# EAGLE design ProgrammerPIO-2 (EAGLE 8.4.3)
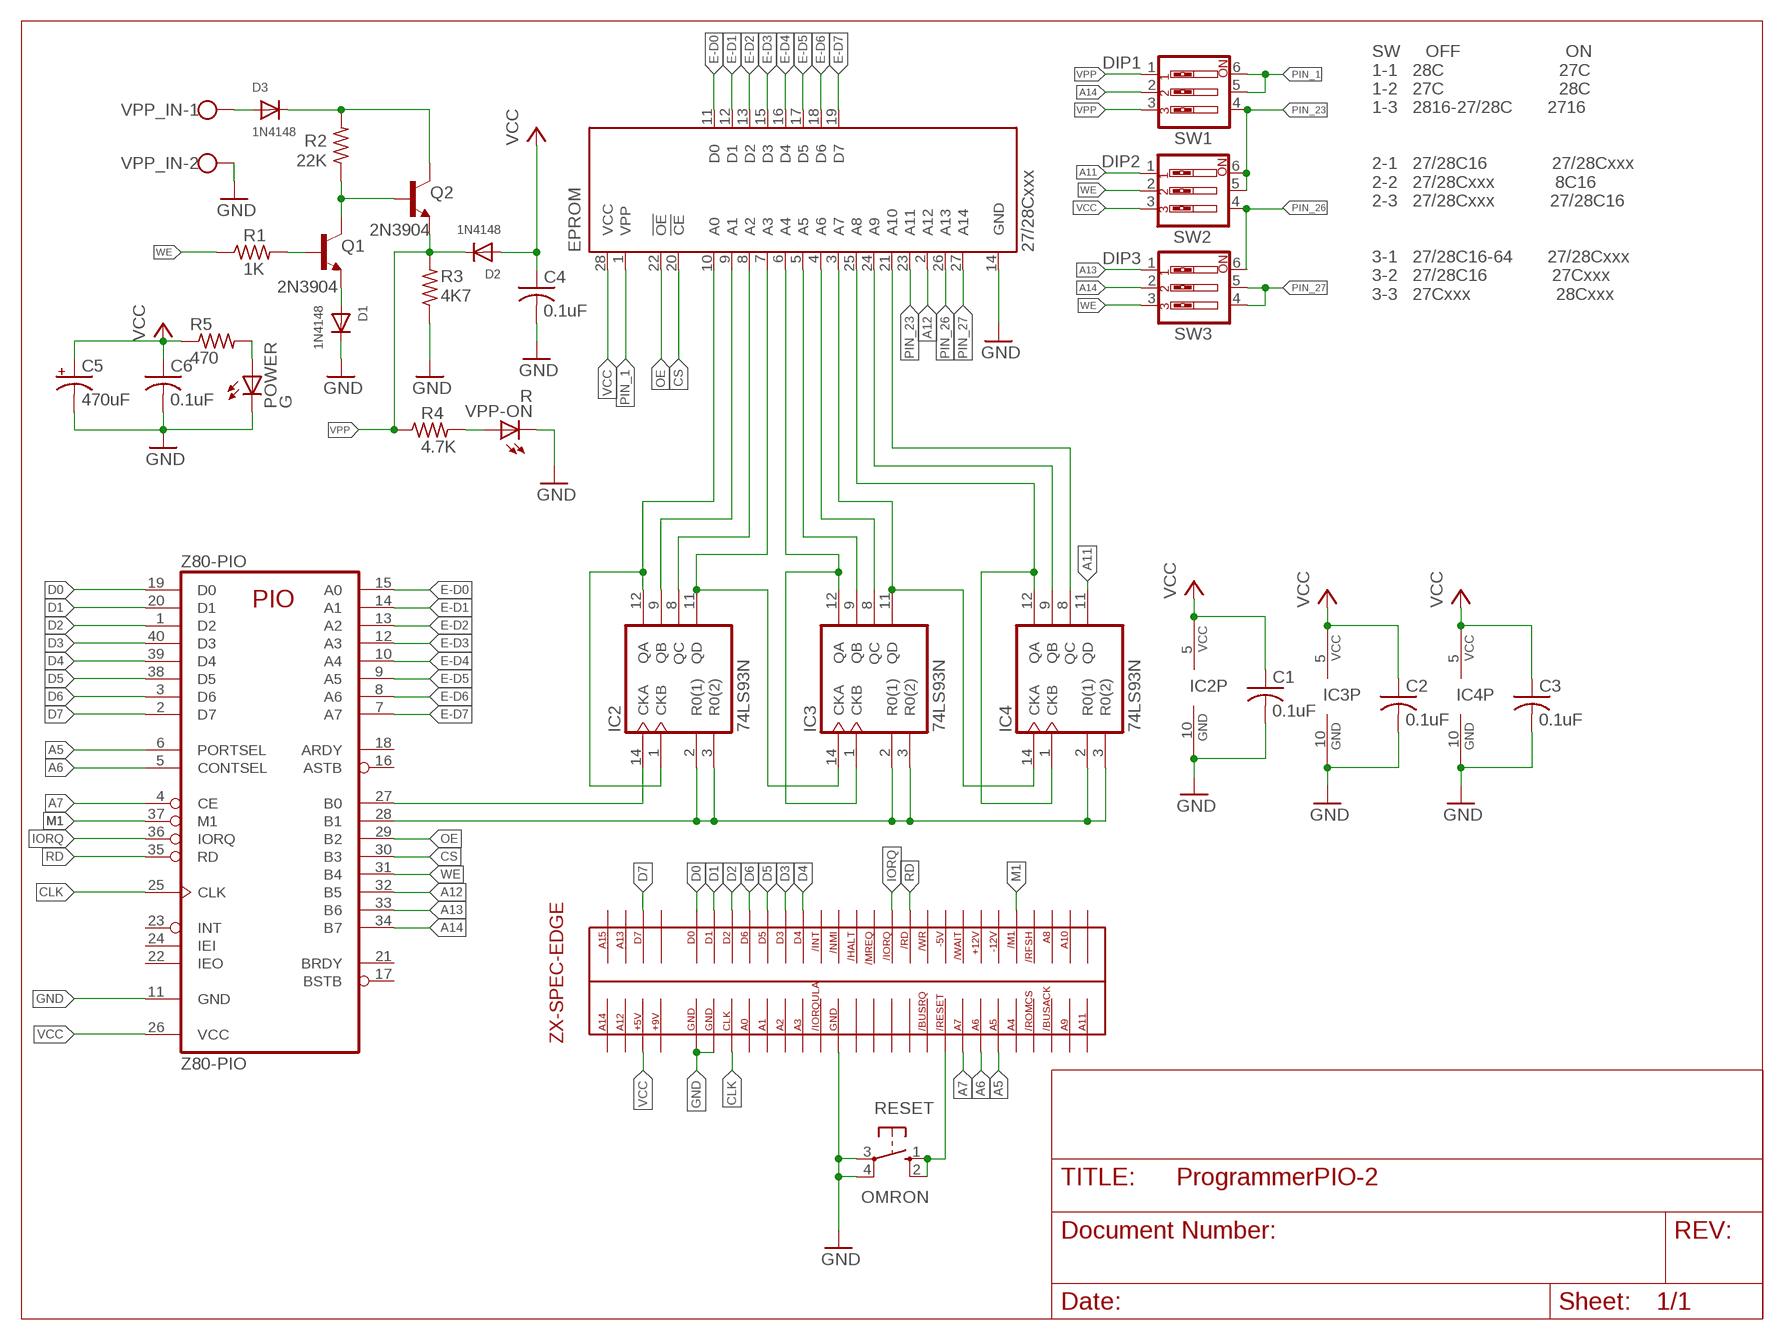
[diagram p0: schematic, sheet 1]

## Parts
1  ZX-EDGE-SPECCY  [ZX-EDGE-SPEC]
C1  0.1uF  C-US025-025X050  [C025-025X050]
C2  0.1uF  C-US025-025X050  [C025-025X050]
C3  0.1uF  C-US025-025X050  [C025-025X050]
C4  0.1uF  C-US025-025X050  [C025-025X050]
C5  470uF  CPOL-USE2.5-5  [E2,5-5]
C6  0.1uF  C-US025-025X050  [C025-025X050]
D1  1N4148  DIODEDO-1N4148  [DO-1N4148]
D2  1N4148  DIODEDO-1N4148  [DO-1N4148]
D3  1N4148  DIODEDO-1N4148  [DO-1N4148]
EPROM  27/28Cxxx  27C256P  [DIL28-6]
IC2  74LS93N  [DIL14]
IC3  74LS93N  [DIL14]
IC4  74LS93N  [DIL14]
POWER  G  LED5MM  [LED5MM]
Q1  2N3904  [TO92]
Q2  2N3904  [TO92]
R1  1K  R-US_0204/7  [0204/7]
R2  22K  R-US_0204/7  [0204/7]
R3  4K7  R-US_0204/7  [0204/7]
R4  4.7K  R-US_0204/7  [0204/7]
R5  470  R-US_0204/7  [0204/7]
RESET  OMRON  10-XX  [B3F-10XX]
SW1  DIP1  SW_DIP-3  [EDG-03]
SW2  DIP2  SW_DIP-3  [EDG-03]
SW3  DIP3  SW_DIP-3  [EDG-03]
VPP-ON  R  LED5MM  [LED5MM]
VPP_IN  W237-102  [W237-102]
Z80-PIO  Z80-PIO  Z80PIO  [DIL40]

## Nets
A5: 1.A5 Z80-PIO.6(PORTSEL)
A6: 1.A6 Z80-PIO.5(CONTSEL)
A7: 1.A7 Z80-PIO.4(CE)
A11: IC4.11(QD) SW2.1
A12: EPROM.2(A12) Z80-PIO.32(B5)
A13: SW3.1 Z80-PIO.33(B6)
A14: SW1.2 SW3.2 Z80-PIO.34(B7)
B0: IC2.14(CKA) Z80-PIO.27(B0)
B1: IC2.2(R0(1)) IC2.3(R0(2)) IC3.2(R0(1)) IC3.3(R0(2)) IC4.2(R0(1)) IC4.3(R0(2)) Z80-PIO.28(B1)
CLK: 1.CLK Z80-PIO.25(CLK)
CS: EPROM.20(!CE) Z80-PIO.30(B3)
D0: 1.D0 Z80-PIO.19(D0)
D1: 1.D1 Z80-PIO.20(D1)
D2: 1.D2 Z80-PIO.1(D2)
D3: 1.D3 Z80-PIO.40(D3)
D4: 1.D4 Z80-PIO.39(D4)
D5: 1.D5 Z80-PIO.38(D5)
D6: 1.D6 Z80-PIO.3(D6)
D7: 1.D7 Z80-PIO.2(D7)
E-D0: EPROM.11(D0) Z80-PIO.15(A0)
E-D1: EPROM.12(D1) Z80-PIO.14(A1)
E-D2: EPROM.13(D2) Z80-PIO.13(A2)
E-D3: EPROM.15(D3) Z80-PIO.12(A3)
E-D4: EPROM.16(D4) Z80-PIO.10(A4)
E-D5: EPROM.17(D5) Z80-PIO.9(A5)
E-D6: EPROM.18(D6) Z80-PIO.8(A6)
E-D7: EPROM.19(D7) Z80-PIO.7(A7)
GND: 1.GND1 1.GND2 1.GND3 C1.2 C2.2 C3.2 C4.2 C5.- C6.2 D1.C EPROM.14(GND) IC2.10(GND) IC3.10(GND) IC4.10(GND) POWER.K(C) R3.1 RESET.3(P) RESET.4(P1) VPP-ON.K(C) VPP_IN.2 Z80-PIO.11(GND)
IORQ: 1./IORQ Z80-PIO.36(IORQ)
M1: 1./M1 Z80-PIO.37(M1)
N$1: EPROM.10(A0) IC2.1(CKB) IC2.12(QA)
N$2: EPROM.9(A1) IC2.9(QB)
N$3: EPROM.8(A2) IC2.8(QC)
N$4: EPROM.7(A3) IC2.11(QD) IC3.14(CKA)
N$5: EPROM.6(A4) IC3.1(CKB) IC3.12(QA)
N$6: EPROM.5(A5) IC3.9(QB)
N$7: EPROM.4(A6) IC3.8(QC)
N$8: EPROM.3(A7) IC3.11(QD) IC4.14(CKA)
N$9: EPROM.25(A8) IC4.1(CKB) IC4.12(QA)
N$10: EPROM.24(A9) IC4.9(QB)
N$11: EPROM.21(A10) IC4.8(QC)
N$13: Q1.2(B) R1.2
N$14: D1.A Q1.3(E)
N$15: Q1.1(C) Q2.2(B) R2.1
N$16: D3.A VPP_IN.1
N$17: D3.C Q2.1(C) R2.2
N$18: R4.2 VPP-ON.A
N$19: 1./RST RESET.1(S) RESET.2(S1)
N$20: POWER.A R5.2
OE: EPROM.22(!OE) Z80-PIO.29(B2)
PIN_1: EPROM.1(VPP) SW1.5 SW1.6
PIN_23: EPROM.23(A11) SW1.4 SW2.5 SW2.6
PIN_26: EPROM.26(A13) SW2.4 SW3.6
PIN_27: EPROM.27(A14) SW3.4 SW3.5
RD: 1./RD Z80-PIO.35(RD)
VCC: 1.+5 C1.1 C2.1 C3.1 C4.1 C5.+ C6.1 D2.A EPROM.28(VCC) IC2.5(VCC) IC3.5(VCC) IC4.5(VCC) R5.1 SW2.3 Z80-PIO.26(VCC)
VPP: D2.C Q2.3(E) R3.2 R4.1 SW1.1 SW1.3
WE: R1.1 SW2.2 SW3.3 Z80-PIO.31(B4)
Unconnected: 1.+9 1.+12 1.-5(-5V) 1.-12 1./BUSAK 1./BUSRQ 1./HALT 1./INT 1./IORQULA 1./MREQ 1./NMI 1./RFSH(/REFSH) 1./ROMCS 1./WAIT 1./WR 1.A0 1.A1 1.A2 1.A3 1.A4 1.A8 1.A9 1.A10 1.A11 1.A12 1.A13 1.A14 1.A15 1.N/C1 1.N/C2 1.N/C3 1.N/C4 1.N/C5 1.N/C6 Z80-PIO.16(ASTB) Z80-PIO.17(BSTB) Z80-PIO.18(ARDY) Z80-PIO.21(BRDY) Z80-PIO.22(IEO) Z80-PIO.23(INT) Z80-PIO.24(IEI)

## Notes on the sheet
- SW     OFF                     ON
  1-1   28C                       27C
  1-2   27C                       28C
  1-3   2816-27/28C       2716
  
  
  2-1   27/28C16             27/28Cxxx
  2-2   27/28Cxxx            8C16
  2-3   27/28Cxxx           27/28C16
  
  
  3-1   27/28C16-64       27/28Cxxx
  3-2   27/28C16             27Cxxx
  3-3   27Cxxx                 28Cxxx

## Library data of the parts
1 = sinclair-zx-spec:ZX-EDGE-SPECCY: ZX SPECTRUM EDGE CONNECTOR
C1-C4 C6 = rcl:C-US: CAPACITOR, American symbol
C5 = rcl:CPOL-US: POLARIZED CAPACITOR, American symbol
D1-D3 = adafruit:DIODE: Diode
EPROM = microchip:27*256: CMOS EPROM 256 K (32 K x 8), low voltage; MF: Arrow Electronics; MPN: M27C256B15F1; OC_FARNELL: 1125431; OC_NEWARK: 93K7335
IC2-IC4 = 74xx-us:74*93: Decade, divide by twelve and binary COUNTER
POWER = adafruit:LED: LED
Q1 Q2 = transistor-npn:2N3904: NPN Transistor
R1-R5 = rcl:R-US_: RESISTOR, American symbol
RESET = switch-omron:10-XX: OMRON SWITCH; MPN: B3F-1000; OC_FARNELL: 176432; OC_NEWARK: 36M3542
SW1-SW3 = special:SW_DIP-3: DIP SWITCH
VPP-ON = led:LED: LED
VPP_IN = con-wago-500:W237-102: WAGO SCREW CLAMP; MPN: 237-102; OC_FARNELL: unknown; OC_NEWARK: 70K9898
Z80-PIO = zilog:Z80PIO: Z80 FAMILY DEVICE

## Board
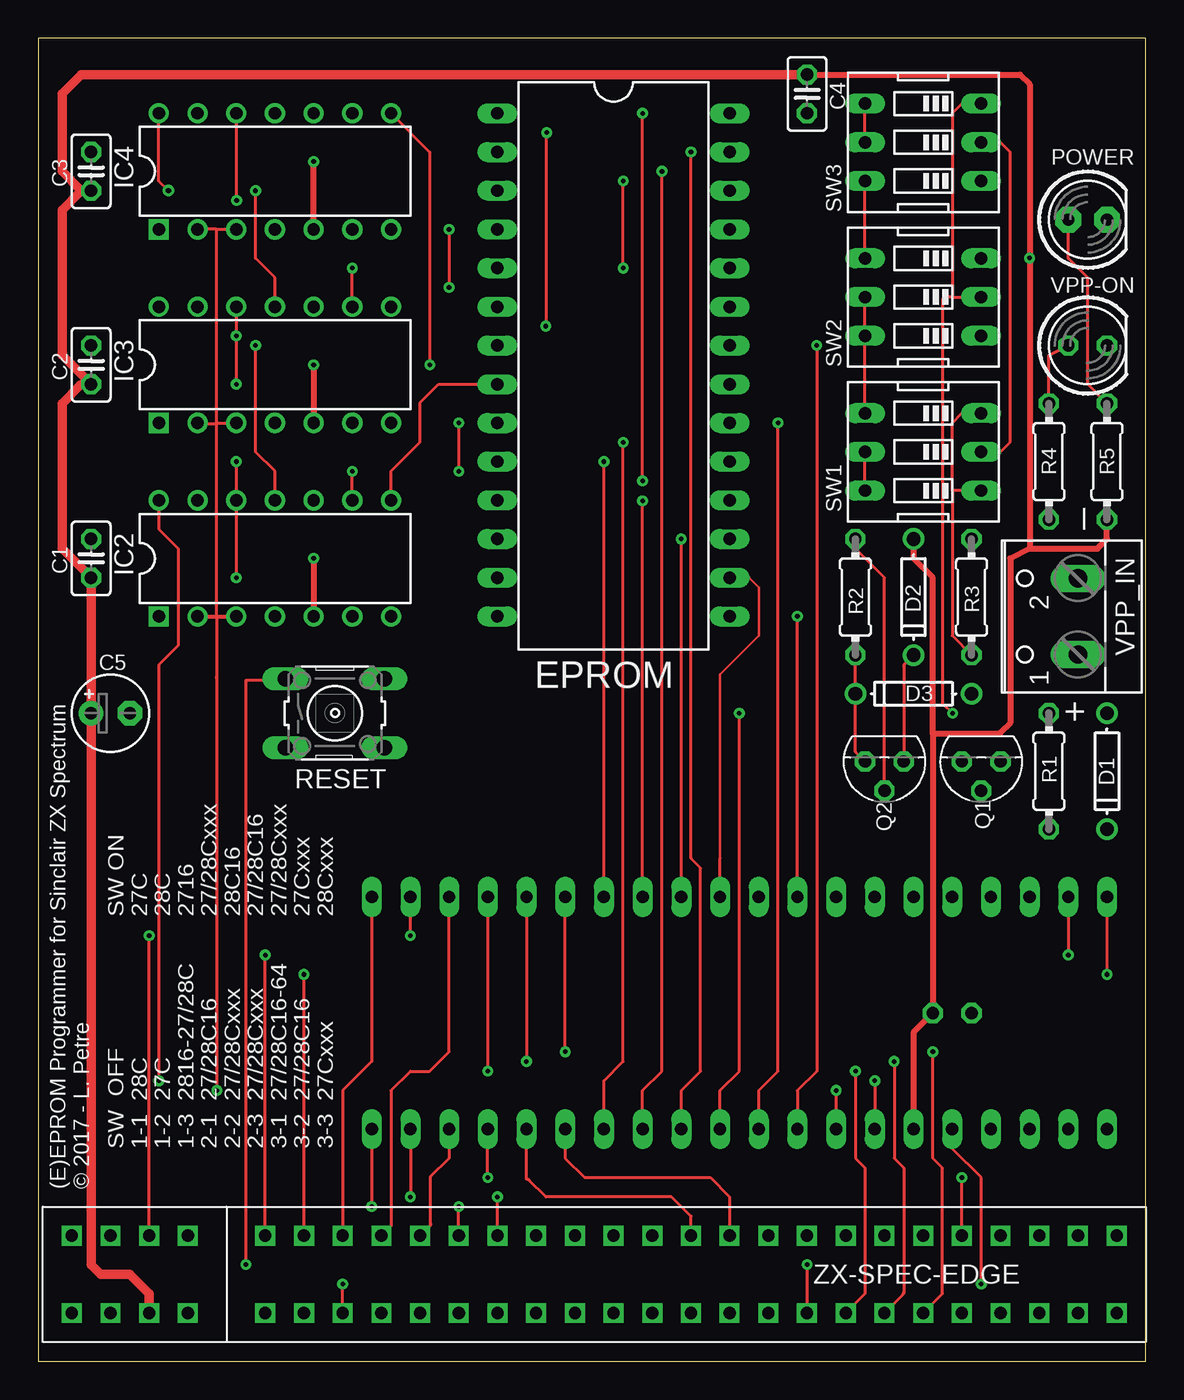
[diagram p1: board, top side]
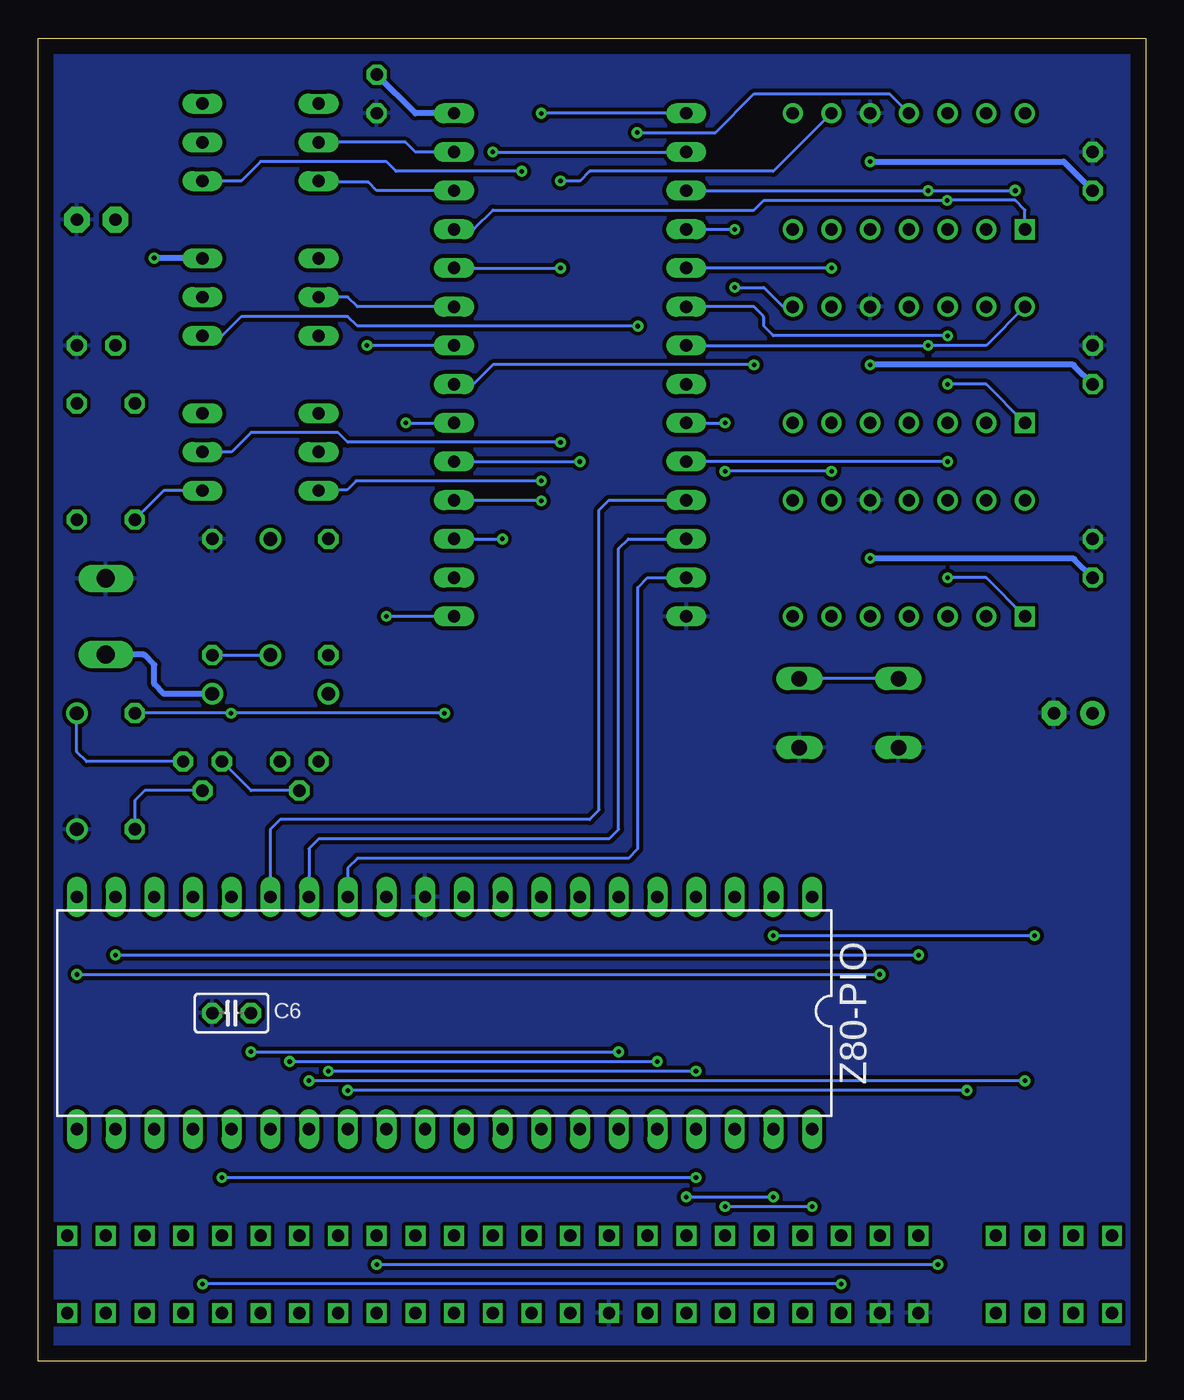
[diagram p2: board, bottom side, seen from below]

Size 72.7 x 86.85 mm. Coordinates in mm from the lower left corner, seen from the top.
Outline: 72.7,0 72.7,86.85 0,86.85 0,0 72.7,0
Copper layers (1*16): Top 0.035mm / dielectric 1.5mm / Bottom 0.035mm
Design rules "default *": minimum track width 6mil, minimum drill 0.3mm, track to track 6mil, track to pad 6mil, pad to pad 6mil, via to via 6mil, smd to smd 6mil, copper to edge 40mil, drill to drill 6mil, minimum pad ring 10mil, minimum via ring 8mil, stop-mask expansion 4mil, vias tented up to drill 0mil, thermal gap 10mil

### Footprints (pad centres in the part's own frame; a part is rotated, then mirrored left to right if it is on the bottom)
ZX-EDGE-SPEC = drill 0.8 square: +5 -5.08,-2.54; +9 -2.54,-2.54; +12 43.18,2.54; -5 38.1,2.54; -12 45.72,2.54; /BUSAK 53.34,-2.54; /BUSRQ 35.56,-2.54; /HALT 25.4,2.54; /INT 20.32,2.54; /IORQ 30.48,2.54; /IORQULA 20.32,-2.54; /M1 48.26,2.54; /MREQ 27.94,2.54; /NMI 22.86,2.54; /RD 33.02,2.54; /RFSH 50.8,2.54; /ROMCS 50.8,-2.54; /RST 38.1,-2.54; /WAIT 40.64,2.54; /WR 35.56,2.54; A0 10.16,-2.54; A1 12.7,-2.54; A2 15.24,-2.54; A3 17.78,-2.54; A4 48.26,-2.54; A5 45.72,-2.54; A6 43.18,-2.54; A7 40.64,-2.54; A8 53.34,2.54; A9 55.88,-2.54; A10 55.88,2.54; A11 58.42,-2.54; A12 -7.62,-2.54; A13 -7.62,2.54; A14 -10.16,-2.54; A15 -10.16,2.54; CLK 7.62,-2.54; D0 2.54,2.54; D1 5.08,2.54; D2 7.62,2.54; D3 15.24,2.54; D4 17.78,2.54; D5 12.7,2.54; D6 10.16,2.54; D7 -5.08,2.54; GND1 2.54,-2.54; GND2 5.08,-2.54; GND3 22.86,-2.54; N/C1 -2.54,2.54; N/C2 58.42,2.54; N/C3 25.4,-2.54; N/C4 27.94,-2.54; N/C5 30.48,-2.54; N/C6 33.02,-2.54
C025-025X050 = drill 0.813 octagon: 1 -1.27,0; 2 1.27,0
E2,5-5 = drill 0.813 pad 1.6: + -1.27,0 | drill 0.813 pad 1.6 octagon: - 1.27,0
DO-1N4148 = drill 0.9: A -3.81,0; C 3.81,0
DIL28-6 = drill 0.813 long: 1 -16.51,-7.62; 2 -13.97,-7.62; 3 -11.43,-7.62; 4 -8.89,-7.62; 5 -6.35,-7.62; 6 -3.81,-7.62; 7 -1.27,-7.62; 8 1.27,-7.62; 9 3.81,-7.62; 10 6.35,-7.62; 11 8.89,-7.62; 12 11.43,-7.62; 13 13.97,-7.62; 14 16.51,-7.62; 15 16.51,7.62; 16 13.97,7.62; 17 11.43,7.62; 18 8.89,7.62; 19 6.35,7.62; 20 3.81,7.62; 21 1.27,7.62; 22 -1.27,7.62; 23 -3.81,7.62; 24 -6.35,7.62; 25 -8.89,7.62; 26 -11.43,7.62; 27 -13.97,7.62; 28 -16.51,7.62
DIL14 = drill 0.813 square: 1 -7.62,-3.81 | drill 0.813: 2 -5.08,-3.81; 3 -2.54,-3.81; 4 0,-3.81; 5 2.54,-3.81; 6 5.08,-3.81; 7 7.62,-3.81; 8 7.62,3.81; 9 5.08,3.81; 10 2.54,3.81; 11 0,3.81; 12 -2.54,3.81; 13 -5.08,3.81; 14 -7.62,3.81
LED5MM = drill 0.813 pad 1.676 octagon: A -1.27,0; K 1.27,0
TO92 = drill 0.813 octagon: 1 1.27,0; 2 0,1.905; 3 -1.27,0
0204/7 = drill 0.813 octagon: 1 -3.81,0; 2 3.81,0
B3F-10XX = drill 1.016 long: 1 -3.251,2.261; 2 3.251,2.261; 3 -3.251,-2.261; 4 3.251,-2.261
EDG-03 = drill 0.813 long: 1 -2.54,-3.81; 2 0,-3.81; 3 2.54,-3.81; 4 2.54,3.81; 5 0,3.81; 6 -2.54,3.81
LED5MM' = drill 0.813 octagon: A -1.27,0; K 1.27,0
W237-102 = drill 1.194 long: 1 -2.5,-1.27; 2 2.5,-1.27
DIL40 = drill 0.813 long: 1 -24.13,-7.62; 2 -21.59,-7.62; 3 -19.05,-7.62; 4 -16.51,-7.62; 5 -13.97,-7.62; 6 -11.43,-7.62; 7 -8.89,-7.62; 8 -6.35,-7.62; 9 -3.81,-7.62; 10 -1.27,-7.62; 11 1.27,-7.62; 12 3.81,-7.62; 13 6.35,-7.62; 14 8.89,-7.62; 15 11.43,-7.62; 16 13.97,-7.62; 17 16.51,-7.62; 18 19.05,-7.62; 19 21.59,-7.62; 20 24.13,-7.62; 21 24.13,7.62; 22 21.59,7.62; 23 19.05,7.62; 24 16.51,7.62; 25 13.97,7.62; 26 11.43,7.62; 27 8.89,7.62; 28 6.35,7.62; 29 3.81,7.62; 30 1.27,7.62; 31 -1.27,7.62; 32 -3.81,7.62; 33 -6.35,7.62; 34 -8.89,7.62; 35 -11.43,7.62; 36 -13.97,7.62; 37 -16.51,7.62; 38 -19.05,7.62; 39 -21.59,7.62; 40 -24.13,7.62

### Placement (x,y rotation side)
1  12.37,5.71 0 top
C1  3.48,52.7 90 top
C2  3.48,65.41 90 top
C3  3.48,78.11 90 top
C4  50.47,83.19 270 top
C5  4.75,42.55 0 top
C6  60,22.86 180 bottom
D1  70.16,38.73 270 top
D2  57.45,50.16 270 top
D3  57.45,43.81 180 top
EPROM  37.77,65.41 270 top
IC2  15.54,52.7 0 top
IC3  15.54,65.41 0 top
IC4  15.54,78.11 0 top
POWER  68.89,74.93 0 top
Q1  61.9,39.37 180 top
Q2  55.55,39.37 180 top
R1  66.34,38.73 270 top
R2  53.65,50.16 270 top
R3  61.27,50.16 270 top
R4  66.34,59.05 90 top
R5  70.16,59.05 90 top
RESET  19.48,42.55 0 top
SW1  58.09,59.69 90 top
SW2  58.09,69.85 90 top
SW3  58.09,80.01 90 top
VPP-ON  R  [LED5MM']  68.89,66.67 0 top
VPP_IN  66.98,48.9 90 top
Z80-PIO  46.02,22.86 180 bottom

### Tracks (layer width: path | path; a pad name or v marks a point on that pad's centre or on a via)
A5  (via drill 0.3)
  Top 0.2: v34.59,20.32 Z80-PIO.6 | 1.A5 59.36,4.45 59.36,12.7 58.73,13.34 v58.73,20.32
  Bottom 0.2: v58.73,20.32 v34.59,20.32
A6  (via drill 0.3)
  Top 0.2: Z80-PIO.5 v32.05,19.68 | 56.82,4.55 arc-45 56.75,4.37 | 1.A6 56.75,4.37 | 56.75,4.37 arc45 56.82,4.55 | v56.19,19.68 56.19,13.34 56.82,12.7 56.82,4.55
  Bottom 0.2: v56.19,19.68 v32.05,19.68
A7  (via drill 0.3)
  Top 0.2: v53.65,19.05 53.65,13.34 54.28,12.7 54.28,4.45 1.A7 | Z80-PIO.4 v29.52,19.05
  Bottom 0.2: v29.52,19.05 v53.65,19.05
A11  (via drill 0.3)
  Top 0.2: v33.38,80.64 arc45 33.33,80.51 v33.33,67.94
  Bottom 0.2: 33.33,80.64 v33.38,80.64 28.25,80.64 25.71,83.19 16.82,83.19 IC4.11 | v33.33,67.94 51.74,67.94 52.38,68.58 59.36,68.58 60.63,67.31 SW2.1
A12  (via drill 0.3)
  Top 0.2: Z80-PIO.32 42.22,17.78 43.48,19.05 43.48,32.38 42.85,33.02 v42.85,79.38
  Bottom 0.2: v42.85,79.38 EPROM.2
A13  (via drill 0.3)
  Top 0.2: Z80-PIO.33 39.68,17.78 40.95,19.05 v40.95,78.11
  Bottom 0.2: SW3.1 59.36,77.47 58.09,78.74 49.84,78.74 49.2,78.11 v40.95,78.11
A14  (via drill 0.3)
  Top 0.2: Z80-PIO.34 37.14,18.41 38.41,19.68 v38.41,60.33 | SW1.2 63.17,59.69 63.81,60.33 63.81,79.38 63.17,80.01 SW3.2
  Bottom 0.2: v38.41,60.33 52.38,60.33 53.01,60.96 58.73,60.96 60,59.69 SW1.2
B0  (via drill 0.3)
  Top 0.2: IC2.14 7.93,54.61 9.2,53.34 9.2,46.99 7.93,45.72 v7.93,18.41 | v54.91,18.41 Z80-PIO.27
  Bottom 0.2: v7.93,18.41 v54.91,18.41
B1  (via drill 0.3)
  Top 0.2: 11.73,44.78 11.73,44.98 | 11.73,44.78 v11.73,17.78 | v52.38,17.78 Z80-PIO.28 | 11.73,61.56 11.73,48.9 11.73,44.78 | 11.73,61.56 11.73,74.3 | 11.73,74.3 IC4.2 | 11.73,74.3 IC4.3 | IC3.2 arc45 10.54,61.56 11.73,61.56 | 11.73,61.56 arc-45 11.81,61.59 IC3.3
  Top 0.254: IC2.2 11.73,48.9 IC2.3
  Bottom 0.2: v11.73,17.78 v52.38,17.78
CLK  (via drill 0.3)
  Top 0.2: 1.CLK v19.99,5.08 | Z80-PIO.25 60,13.99 arc45 60.01,13.95 61.9,12.06 v61.9,5.08
  Bottom 0.2: v19.99,5.08 v61.9,5.08
CS  (via drill 0.3)
  Top 0.2: Z80-PIO.30 47.3,17.78 48.57,19.05 v48.57,61.59
  Bottom 0.2: v48.57,61.59 EPROM.20
D0  (via drill 0.3)
  Top 0.2: 1.D0 v14.91,26.67 | Z80-PIO.19 v67.61,26.67
  Bottom 0.2: v67.61,26.67 v14.91,26.67
D1  (via drill 0.3)
  Top 0.2: 1.D1 v17.45,25.4 | Z80-PIO.20 v70.16,25.4
  Bottom 0.2: v70.16,25.4 v17.45,25.4
D2
  Top 0.2: Z80-PIO.1 21.9,19.68 19.99,17.78 1.D2
D3  (via drill 0.3)
  Top 0.2: 1.D3 v27.61,10.16 | Z80-PIO.40 v21.9,10.16
  Bottom 0.2: v21.9,10.16 v27.61,10.16
D4  (via drill 0.3)
  Top 0.2: Z80-PIO.39 v24.44,10.79 | 1.D4 v30.15,10.79
  Bottom 0.2: v30.15,10.79 v24.44,10.79
D5
  Top 0.2: Z80-PIO.38 26.98,13.34 25.77,12.13 25.77,9.06 arc-45 25.71,8.89 1.D5
D6
  Top 0.2: 1.D6 23.17,8.89 23.17,17.78 24.44,19.05 25.71,19.05 26.98,20.32 Z80-PIO.3
D7  (via drill 0.3)
  Top 0.2: 1.D7 v7.29,27.94 | v24.44,27.94 Z80-PIO.2
  Bottom 0.2: v7.29,27.94 v24.44,27.94
E-D0
  Bottom 0.2: EPROM.11 35.23,56.52 35.87,55.88 35.87,36.2 36.5,35.56 56.82,35.56 57.45,34.92 Z80-PIO.15
E-D1
  Bottom 0.2: EPROM.12 33.96,53.98 34.59,53.34 34.59,34.92 35.23,34.29 54.28,34.29 54.91,33.66 Z80-PIO.14
E-D2
  Bottom 0.2: EPROM.13 32.69,51.44 33.33,50.8 33.33,33.66 33.96,33.02 51.74,33.02 52.38,32.38 Z80-PIO.13
E-D3  (via drill 0.3)
  Top 0.2: Z80-PIO.12 v49.84,48.9
  Bottom 0.2: EPROM.15 v49.84,48.9
E-D4
  Top 0.152: 44.76,33.02 44.76,45.09 47.3,47.62 47.3,50.8 46.66,51.44 EPROM.16
  Top 0.2: Z80-PIO.10 44.76,33.02
E-D5  (via drill 0.3)
  Top 0.2: Z80-PIO.9 v42.22,53.98
  Bottom 0.2: EPROM.17 v42.22,53.98
E-D6  (via drill 0.3)
  Top 0.2: Z80-PIO.8 v39.68,56.48 39.68,56.52
  Bottom 0.2: EPROM.18 39.68,56.52 v39.68,56.48
E-D7  (via drill 0.3)
  Top 0.2: Z80-PIO.7 v37.14,59.05
  Bottom 0.2: EPROM.19 v37.14,59.05
GND
  pour Bottom (isolate 0.254): 72.7,0 0.05,-0.13 0.05,86.87 72.82,86.87 72.57,0.13
IORQ
  Top 0.2: Z80-PIO.36 32.05,11.96 arc-45 32.23,11.89 33.33,10.79 41.58,10.79 42.85,9.53 1./IORQ
M1  (via drill 0.3)
  Top 0.2: 1./M1 v60.63,12.06 | v29.52,12.06 Z80-PIO.37
  Bottom 0.2: v60.63,12.06 v29.52,12.06
N$1  (via drill 0.3)
  Top 0.2: v13.01,51.44 13.01,56.4 IC2.12 v13.01,59.05
  Bottom 0.2: 10.46,51.44 v13.01,51.44 | v13.01,59.05 EPROM.10
  Bottom 0.203: IC2.1 10.46,51.44
N$2  (via drill 0.3)
  Top 0.2: IC2.9 v20.62,58.42 | v27.61,61.59 v27.61,58.42
  Bottom 0.2: v20.62,58.42 v27.61,58.42 | EPROM.9 v27.61,61.59
N$3
  Top 0.2: IC2.8 23.17,58.42 25.07,60.33 25.07,62.91 26.3,64.14 EPROM.8
N$4  (via drill 0.3)
  Top 0.2: IC2.11 15.54,58.42 14.28,59.69 v14.28,66.67
  Bottom 0.2: EPROM.7 v14.28,66.67 10.46,66.67
  Bottom 0.203: IC3.14 10.46,66.67
N$5  (via drill 0.3)
  Top 0.2: IC3.12 v13.01,67.31 v13.01,64.14
  Bottom 0.2: 10.46,64.14 v13.01,64.14 | v13.01,67.31 24.44,67.31 25.07,67.94 25.07,68.47 arc-45 25.14,68.65 25.71,69.22 EPROM.6
  Bottom 0.203: IC3.1 10.46,64.14
N$6  (via drill 0.3)
  Top 0.2: IC3.9 v20.62,71.75
  Bottom 0.2: v20.62,71.75 EPROM.5
N$7  (via drill 0.3)
  Top 0.2: v26.98,74.3 v26.98,70.48
  Bottom 0.2: EPROM.4 v26.98,74.3 | v26.98,70.48 25.07,70.48 23.8,69.22 IC3.8
N$8  (via drill 0.3, 0.35)
  Top 0.2: IC3.11 15.54,71.12 14.28,72.39 v14.28,76.83
  Top 0.203: v8.56,76.83 7.93,77.47 IC4.14
  Bottom 0.2: EPROM.3 v14.28,76.83 v8.56,76.83
N$9  (via drill 0.3)
  Top 0.2: IC4.12 13.01,76.23 v13.03,76.2
  Bottom 0.2: EPROM.25 44.23,74.3 arc-45 44.05,74.37 42.85,75.56 25.71,75.56 25.07,76.2 v13.03,76.2
  Bottom 0.203: IC4.1 7.93,75.56 8.56,76.2 v13.03,76.2
N$10  (via drill 0.3)
  Top 0.2: v38.41,71.75 v38.41,77.47
  Bottom 0.2: EPROM.24 v38.41,71.75 | v38.41,77.47 37.14,77.47 36.5,78.11 24.44,78.11 IC4.9
N$11  (via drill 0.3)
  Top 0.2: v25.71,65.41 25.71,79.38 IC4.8
  Bottom 0.2: v25.71,65.41 42.85,65.41 44.12,64.14 EPROM.21
N$13
  Bottom 0.2: Q1.2 65.71,37.47 66.34,36.83 R1.2
N$14
  Bottom 0.2: Q1.3 69.52,39.37 70.16,40.01 D1.A
N$15
  Top 0.2: Q2.2 55.55,51.44 53.65,53.34 R2.1
  Bottom 0.2: Q2.2 58.73,37.47 Q1.1
N$16
  Bottom 0.406: D3.A 64.44,43.81 65.08,44.45 65.08,45.72 65.71,46.35 arc-45 65.81,46.4 VPP_IN.1
N$17
  Top 0.2: Q2.1 53.65,40.01 D3.C R2.2
N$18
  Top 0.203: VPP-ON.A 66.34,66.04 R4.2
N$19  (via drill 0.3)
  Top 0.2: v13.64,6.35 13.64,42.11 | v50.47,6.35 1./RST
  Top 0.203: 13.64,42.11 13.64,44.7 16.13,44.7 RESET.1
  Bottom 0.2: RESET.1 RESET.2 | v13.64,6.35 v50.47,6.35
N$20
  Top 0.203: R5.2 68.89,64.14 68.89,71.12 67.61,72.39 POWER.A
OE  (via drill 0.3)
  Top 0.2: v51.11,66.67 51.11,19.05 49.84,17.78 Z80-PIO.29
  Bottom 0.2: EPROM.22 v51.11,66.67
PIN_1  (via drill 0.3)
  Top 0.2: v39.68,57.78 v39.68,81.92 | SW1.6 SW1.5
  Bottom 0.2: EPROM.1 v39.68,81.92 | v39.68,57.78 51.83,57.78 52.42,57.19 54.24,57.19 SW1.6
PIN_23
  Top 0.2: SW1.4 SW2.6 SW2.5
  Bottom 0.2: EPROM.23 51.74,69.22 52.38,69.85 SW2.5
PIN_26
  Top 0.2: SW2.4 SW3.6
  Bottom 0.2: SW3.6 53.02,77.38 51.02,77.38 50.47,76.83 EPROM.26
PIN_27
  Top 0.2: SW3.5 SW3.4
  Bottom 0.2: EPROM.27 47.93,79.38 48.57,80.01 SW3.5
RD
  Top 0.2: Z80-PIO.35 34.59,13.34 35.87,12.06 44.12,12.06 45.39,10.79 1./RD
VCC  (via drill 0.3)
  Top 0.406: D2.A 57.45,52.7 58.73,51.44 58.73,41.19 | 58.73,41.19 C6.1 57.45,21.59 Z80-PIO.26 | v18.09,65.41 IC3.5 | v18.09,52.7 IC2.5 | C4.1 64.44,84.45 65.08,83.82 v65.08,72.41 65.08,53.34 | 65.08,53.34 69.52,53.34 70.16,53.98 R5.1 | 58.73,41.19 62.98,41.19 arc45 63.16,41.26 63.81,41.91 63.81,52.7 65.08,53.34 | IC4.5 v18.09,78.74
  Top 0.61: 2.95,76.83 arc45 2.77,76.76 1.57,75.56 1.57,66.04 C2.1 2.95,64.14 arc45 2.77,64.06 1.57,62.87 1.57,53.45 arc45 1.65,53.27 C1.1 C5.+ 3.48,6.35 4.12,5.71 6.02,5.71 7.29,4.45 1.+5 | C4.1 2.84,84.45 1.57,83.19 1.57,78.11 2.77,76.91 arc45 2.95,76.83 | 2.95,76.83 C3.1
  Bottom 0.2: 18.05,65.41 v18.09,65.41
  Bottom 0.406: C1.1 4.68,52.63 arc-45 4.85,52.7 v18.09,52.7 | C2.1 4.71,65.36 arc-45 4.81,65.41 18.05,65.41 | EPROM.28 47.93,81.92 C4.1 | SW2.3 65.08,72.39 v65.08,72.41 | v18.09,78.74 5.38,78.74 C3.1
VPP
  Top 0.2: SW1.3 60.63,62.23 60,61.59 60,57.15 60,47.62 R3.2 | D2.C 56.89,45.79 arc45 56.82,45.62 Q2.3
  Top 0.203: SW1.1 60,57.15
  Bottom 0.2: R4.1 64.44,57.15 SW1.1 | R3.2 D2.C
WE  (via drill 0.3)
  Top 0.2: Z80-PIO.31 44.76,17.78 46.02,19.05 v46.02,42.55 | SW3.3 60.63,82.55 60,81.92 60,69.85 | 60.63,69.85 SW2.2 60,69.85 | v60.03,42.55 60,42.55 59.36,43.18 59.36,69.75 59.47,69.85 60,69.85
  Bottom 0.2: v46.02,42.55 v60.03,42.55 R1.1

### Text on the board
tNames: _ | + | SW ON / 27C / 28C / 2716 / 27/28Cxxx / 28C16 / 27/28C16 / 27/28Cxxx / 27Cxxx / 28Cxxx | SW OFF / 1-1 28C / 1-2 27C / 1-3 2816-27/28C / 2-1 27/28C16 / 2-2 27/28Cxxx / 2-3 27/28Cxxx / 3-1 27/28C16-64 / 3-2 27/28C16 / 3-3 27Cxxx | (E)EPROM Programmer for Sinclair ZX Spectrum / © 2017 - L. Petre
